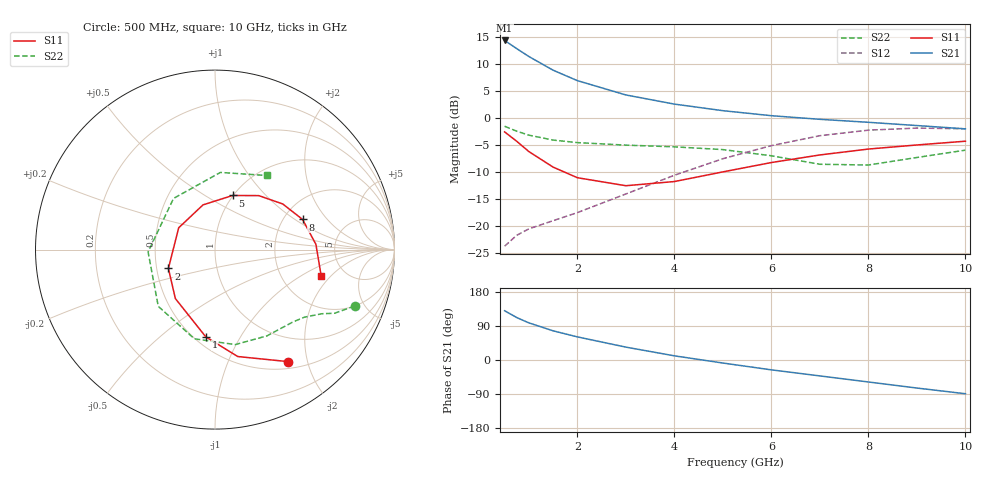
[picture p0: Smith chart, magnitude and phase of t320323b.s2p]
!AT-32032
!S-PARAMETERS at Vce=2.7V  Ic=2mA.  LAST UPDATED 05-29-98
# ghz s ma r 50
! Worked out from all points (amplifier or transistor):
!   13 points, 500 MHz to 10 GHz, reference 50 ohm
!   highest |S21| = 14.4 dB at 500 MHz (marker M1)
!   |S21| within 3 dB of that: start of sweep to 1.005 GHz
!   unconditionally stable (mu >= 1): 1.78 GHz to 3.203 GHz
!   at 1 GHz: K = 0.72, MSG = 16.0 dB, |S12| = -20.5 dB
!   at 4 GHz: K = 0.91, MSG = 6.6 dB, |S12| = -10.6 dB
!   at 10 GHz: K = 0.97, MSG = 0.0 dB, |S12| = -2.0 dB
!   lowest NFmin = 0.90 dB at 900 MHz
!   S11 on the Smith chart (normalised r, x): 500 MHz: 0.60, -1.68; 1 GHz: 0.57, -0.73; 2 GHz: 0.58, -0.13; 5 GHz: 0.99, +0.67; 8 GHz: 2.53, +1.16; 10 GHz: 3.33, -1.57
0.5  0.744 -57.0  5.232 130.0  0.065 60.0  0.839 -22.0
0.75  0.609 -78.0  4.394 112.0  0.082 52.0  0.755 -28.0
1  0.489 -96.0  3.714 98.0  0.094 49.0  0.694 -31.0
1.5  0.351 -129.0  2.774 77.0  0.112 48.0  0.625 -37.0
2  0.28 -158.0  2.221 61.0  0.133 49.0  0.592 -43.0
3  0.236 149.0  1.636 34.0  0.198 50.0  0.561 -59.0
4  0.258 105.0  1.346 11.0  0.295 44.0  0.541 -78.0
5  0.317 72.0  1.17 -8.0  0.42 30.0  0.51 -103.0
6  0.387 51.0  1.051 -26.0  0.555 13.0  0.447 -135.0
7  0.455 34.0  0.973 -42.0  0.686 -8.0  0.373 -178.0
8  0.516 19.0  0.913 -58.0  0.772 -30.0  0.367 129.0
9  0.563 3.0  0.852 -74.0  0.807 -52.0  0.431 86.0
10  0.61 -14.0  0.794 -89.0  0.795 -73.0  0.504 55.0
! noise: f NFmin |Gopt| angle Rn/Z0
0.9  0.9  0.38  57  0.21
1.8  1.2  0.41  124  0.12
2  1.2  0.42  136  0.11
2.5  1.4  0.44  176  0.07
3  1.6  0.47  -152  0.1
3.5  1.8  0.52  -123  0.21
4  2.1  0.57  -100  0.41
